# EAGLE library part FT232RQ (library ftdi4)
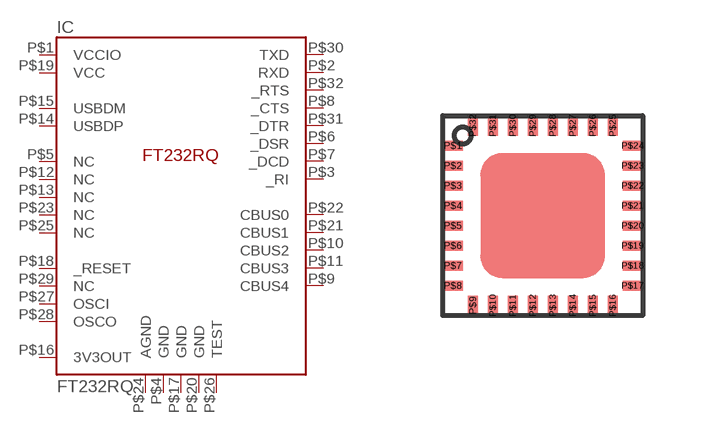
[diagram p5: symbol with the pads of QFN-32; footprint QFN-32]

Designator prefix IC

## FT232RQ  [QFN-32]
P$1  VCCIO  pwr
P$2  RXD  in
P$3  _RI  in
P$4  GND  pwr
P$5  NC  nc
P$6  _DSR  in
P$7  _DCD  in
P$8  _CTS  in
P$9  CBUS4
P$10  CBUS2
P$11  CBUS3
P$12  NC  nc
P$13  NC  nc
P$14  USBDP
P$15  USBDM
P$16  3V3OUT  out
P$17  GND  pwr
P$18  _RESET  in
P$19  VCC  pwr
P$20  GND  pwr
P$21  CBUS1
P$22  CBUS0
P$23  NC  nc
P$24  AGND  pwr
P$25  NC  nc
P$26  TEST
P$27  OSCI  in
P$28  OSCO  out
P$29  NC  nc
P$30  TXD  out
P$31  _DTR  in
P$32  _RTS  out

## Footprint QFN-32 (pad centres in mm)
QFN-32 package (5mm x 5mm)
smd 0.5 x 0.25: P$1 0.25,-0.75; P$2 0.25,-1.25; P$3 0.25,-1.75; P$4 0.25,-2.25; P$5 0.25,-2.75; P$6 0.25,-3.25; P$7 0.25,-3.75; P$8 0.25,-4.25; P$17 4.75,-4.25; P$18 4.75,-3.75; P$19 4.75,-3.25; P$20 4.75,-2.75; P$21 4.75,-2.25; P$22 4.75,-1.75; P$23 4.75,-1.25; P$24 4.75,-0.75
smd 0.25 x 0.5: P$9 0.75,-4.75; P$10 1.25,-4.75; P$11 1.75,-4.75; P$12 2.25,-4.75; P$13 2.75,-4.75; P$14 3.25,-4.75; P$15 3.75,-4.75; P$16 4.25,-4.75; P$25 4.25,-0.25; P$26 3.75,-0.25; P$27 3.25,-0.25; P$28 2.75,-0.25; P$29 2.25,-0.25; P$30 1.75,-0.25; P$31 1.25,-0.25; P$32 0.75,-0.25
